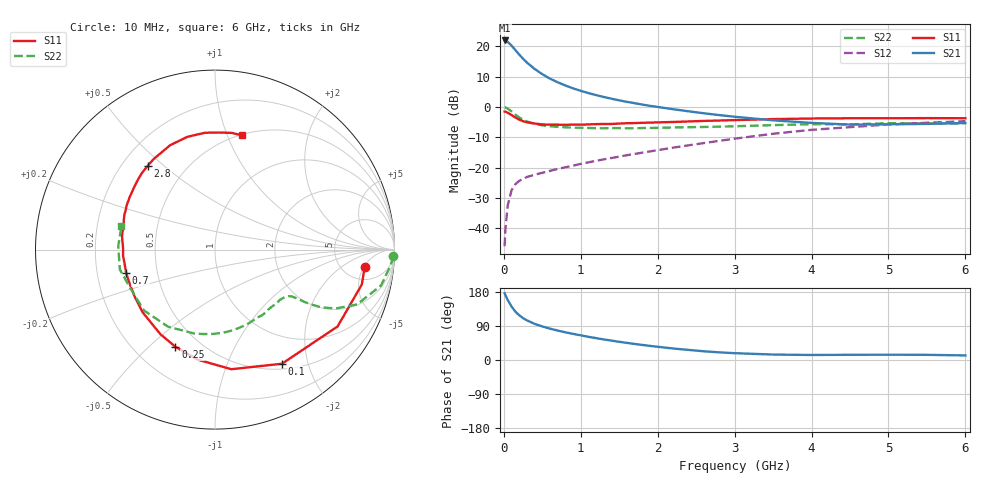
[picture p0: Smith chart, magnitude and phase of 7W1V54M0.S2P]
! Infineon Technologies  Discrete & RF Semiconductors
! BFS17W
! Si NPN RF Bipolar Junction Transistor in SOT323
! VCE = 1.5 V  IC = 4 mA
! Common Emitter S-Parameters:  August  1999
# GHz  S  MA  R  50
!  f  S11  S21  S12  S22
! GHz  MAG  ANG  MAG  ANG  MAG  ANG  MAG  ANG
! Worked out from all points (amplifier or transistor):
!   36 points, 10 MHz to 6 GHz, reference 50 ohm
!   highest |S21| = 21.9 dB at 10 MHz (marker M1)
!   |S21| within 3 dB of that: start of sweep to 143.9 MHz
!   unconditionally stable (mu >= 1): 576.5 MHz to end of sweep
!   at 250 MHz: K = 0.54, MSG = 19.8 dB, |S12| = -23.7 dB
!   at 1.4 GHz: K = 1.32, MAG = 6.4 dB, |S12| = -16.8 dB
!   at 6 GHz: K = 1.11, MAG = -2.3 dB, |S12| = -4.7 dB
!   S11 on the Smith chart (normalised r, x): 10 MHz: 8.09, -5.22; 100 MHz: 0.57, -1.59; 250 MHz: 0.37, -0.61; 700 MHz: 0.33, -0.12; 2.8 GHz: 0.30, +0.44; 6 GHz: 0.51, +1.13
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0.01  0.8399 -6.5  12.5 176.2  0.0051 88.2  0.9942 -2.1
0.02  0.8408 -13.4  12.47 171.3  0.0095 83.4  0.9826 -5.1
0.05  0.8061 -32.1  11.85 158.5  0.0239 74.4  0.9465 -12.2
0.1  0.7372 -59.6  10.3 141.2  0.0424 61.0  0.8483 -21.1
0.15  0.6727 -82.2  8.666 127.6  0.0536 52.3  0.7486 -26.0
0.2  0.6207 -99.0  7.328 118.0  0.0607 48.5  0.6739 -28.5
0.25  0.5844 -112.2  6.238 110.5  0.0655 44.5  0.6167 -29.7
0.3  0.5611 -122.8  5.409 104.6  0.0704 43.9  0.5791 -30.3
0.4  0.5336 -139.1  4.245 95.4  0.0766 43.0  0.527 -30.9
0.5  0.5184 -149.9  3.477 88.6  0.0826 44.1  0.5006 -31.4
0.6  0.5119 -158.5  2.937 82.7  0.0889 45.6  0.483 -32.5
0.7  0.5119 -165.2  2.56 77.7  0.0956 47.3  0.4713 -34.1
0.9  0.5133 -176.0  2.032 69.0  0.1082 50.1  0.4568 -38.1
1.1  0.5173 175.2  1.697 61.1  0.1227 52.5  0.4519 -43.1
1.3  0.5257 167.7  1.463 54.2  0.1376 54.3  0.447 -48.8
1.6  0.5415 158.7  1.217 45.1  0.1607 56.4  0.4467 -57.7
2.2  0.5674 143.1  0.921 30.4  0.2142 58.6  0.4605 -77.2
2.8  0.5989 128.7  0.737 20.2  0.2771 57.5  0.4748 -97.6
3.5  0.6329 113.3  0.604 14.4  0.3629 52.8  0.5029 -121.3
4.5  0.6534 94.9  0.514 13.7  0.4664 41.1  0.518 -155.0
5.5  0.6569 81.8  0.527 13.6  0.5511 29.6  0.5394 177.9
6  0.6538 76.8  0.546 12.1  0.5847 24.0  0.5373 165.9
